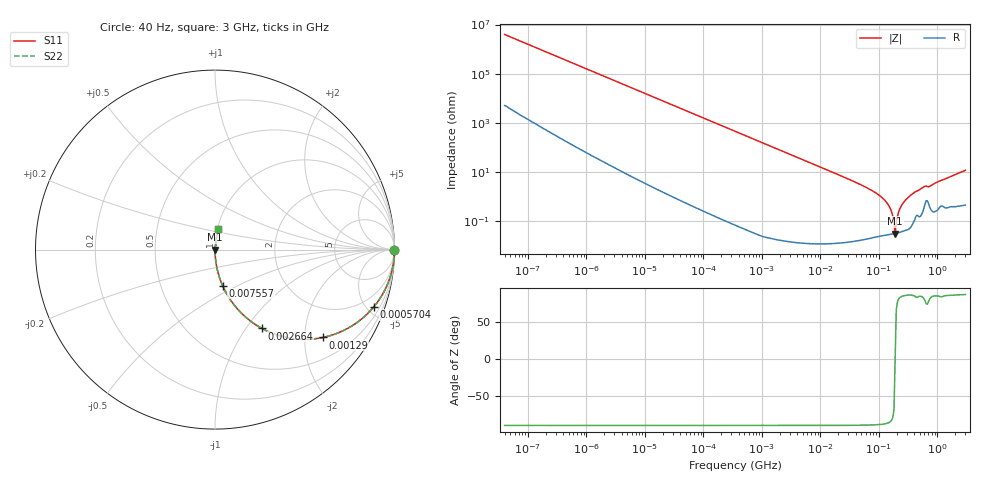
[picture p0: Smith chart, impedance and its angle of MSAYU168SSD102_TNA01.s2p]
! MSAYU168SSD102_TNA01  S-PARAMETER MODEL  ( General Type )
! Model Generated by TAIYO YUDEN Corporation (http://www.ty-top.com)
! Version 2.0
! TAIYO YUDEN Control No. 030711
! Copyright(c) 2003 TAIYO YUDEN CO.,LTD. All Rights Reserved.
! Product Description (link to TY-COMPAS)
! https://ds.yuden.co.jp/TYCOMPAS/or/detail?pn=MSAYU168SSD102KTNA01&u=M
! Products Name : Multilayer Ceramic Capacitors
! Characteristics :
!  Capacitance : 1000 pF , Rated Voltage : 50V
!  Case Size : 1.6 x 0.8 / 0.063 x 0.031 [mm/inch] , Thickness : 0.8 / 0.031 [mm/inch]
!  (Conditions: Temperature = 25 degC , DC Bias Current/Voltage = 0A / 0V)
! External Node Assignments :
!  1  o---| |---o  2
! GND o---------o GND
! Frequency Range : 40Hz  -  3GHz  [ 401 STEP ]
# MHz S RI R 50
! Freq[MHz].  S11 Real  S11 Imag  S21 Real  S21 Imag  S12 Real  S12 Imag  S22 Real  S22 Imag
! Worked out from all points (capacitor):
!   401 points, 40 Hz to 3 GHz, reference 50 ohm
!   read as one part in series: C = 1.01 nF near 44 Hz
!   lowest |Z| = 31.2 mohm at 188.9 MHz (marker M1)
!   series resonance near 189 MHz, so ESL is about 710 pH
!   S11 on the Smith chart (normalised r, x): 40 Hz: open; 570.4 kHz: 1.00, -5.55; 1.29 MHz: 1.00, -2.46; 2.664 MHz: 1.00, -1.19; 7.557 MHz: 1.00, -0.42; 3 GHz: 1.01, +0.23
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4e-05  1 -2.53e-05  3.3e-08 2.53e-05  3.3e-08 2.53e-05  1 -2.53e-05
0.000156  1 -9.85e-05  8.1e-08 9.85e-05  8.1e-08 9.85e-05  1 -9.85e-05
0.000834  1 -0.000527  4.9e-07 0.000527  4.9e-07 0.000527  1 -0.000527
0.017386  0.9999 -0.011  0.000123 0.011  0.000123 0.011  0.9999 -0.011
0.111532  0.9951 -0.0701  0.00495 0.0701  0.00495 0.0701  0.9951 -0.0701
0.362475  0.9502 -0.2175  0.0498 0.2175  0.0498 0.2175  0.9502 -0.2175
0.570368  0.8851 -0.3188  0.1149 0.3188  0.1149 0.3188  0.8851 -0.3188
1.28983  0.6011 -0.4896  0.3989 0.4896  0.3989 0.4896  0.6011 -0.4896
2.664005  0.261 -0.4391  0.739 0.4391  0.739 0.4391  0.261 -0.4391
7.222098  0.0458 -0.2089  0.9542 0.2089  0.9542 0.2089  0.0458 -0.2089
7.557028  0.042 -0.2004  0.958 0.2004  0.958 0.2004  0.042 -0.2004
72.90103  0.000542 -0.0185  0.9995 0.0185  0.9995 0.0185  0.000542 -0.0185
114.7124  0.000326 -0.00871  0.9997 0.00871  0.9997 0.00871  0.000326 -0.00871
150.5692  0.000298 -0.00384  0.9997 0.00384  0.9997 0.00384  0.000298 -0.00384
172.504  0.000302 -0.00154  0.9997 0.00154  0.9997 0.00154  0.000302 -0.00154
188.875  0.000312 -1.31e-05  0.9997 1.31e-05  0.9997 1.31e-05  0.000312 -1.31e-05
206.7996  0.000329 0.00149  0.9997 -0.00149  0.9997 -0.00149  0.000329 0.00149
226.4253  0.000356 0.00307  0.9996 -0.00307  0.9996 -0.00307  0.000356 0.00307
247.9136  0.000396 0.00465  0.9996 -0.00465  0.9996 -0.00465  0.000396 0.00465
372.8114  0.000884 0.0127  0.9991 -0.0127  0.9991 -0.0127  0.000884 0.0127
586.632  0.00397 0.0247  0.996 -0.0247  0.996 -0.0247  0.00397 0.0247
3000  0.0178 0.1143  0.9822 -0.1143  0.9822 -0.1143  0.0178 0.1143
